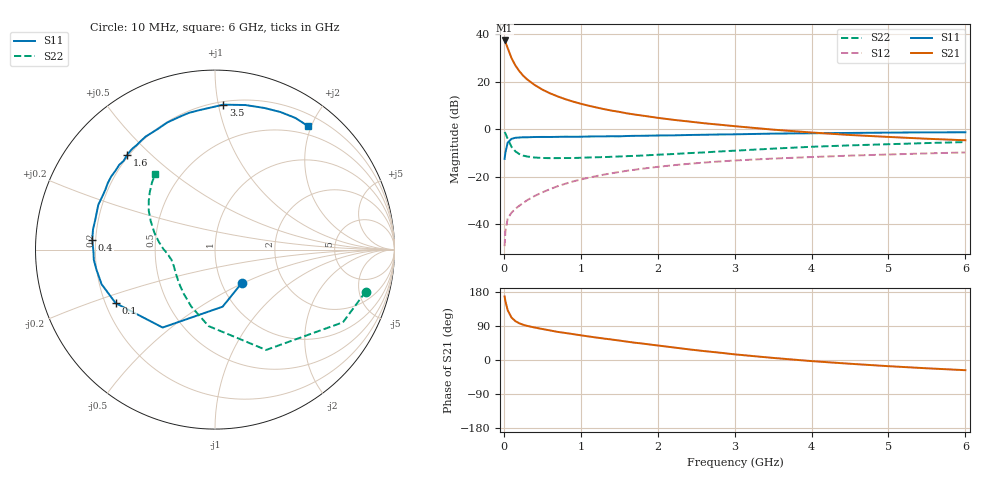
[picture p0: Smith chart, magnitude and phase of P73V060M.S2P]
! SIEMENS Small Signal Semiconductors
! BFP196
! Si NPN RF Bipolar Junction Transistor in SOT143
! VCE = 3 V  IC = 60 mA
! Common Emitter S-Parameters:  May  1996
# GHz  S  MA  R  50
!  f  S11  S21  S12  S22
! GHz  MAG  ANG  MAG  ANG  MAG  ANG  MAG  ANG
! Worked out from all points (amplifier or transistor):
!   36 points, 10 MHz to 6 GHz, reference 50 ohm
!   highest |S21| = 37.3 dB at 10 MHz (marker M1)
!   |S21| within 3 dB of that: start of sweep to 47.61 MHz
!   unconditionally stable (mu >= 1): 413.5 MHz to 4.553 GHz
!   at 250 MHz: K = 0.88, MSG = 26.8 dB, |S12| = -31.0 dB
!   at 1.4 GHz: K = 1.09, MAG = 11.4 dB, |S12| = -18.5 dB
!   at 6 GHz: K = 0.98, MSG = 2.6 dB, |S12| = -9.7 dB
!   S11 on the Smith chart (normalised r, x): 10 MHz: 1.24, -0.49; 100 MHz: 0.24, -0.24; 400 MHz: 0.19, +0.04; 1.6 GHz: 0.19, +0.42; 3.5 GHz: 0.22, +1.03; 6 GHz: 0.37, +1.95
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0.01  0.2386 -51.5  73.17 167.7  0.0035 78.8  0.8715 -15.6
0.02  0.3209 -82.4  67.9 155.5  0.0071 73.5  0.82 -29.6
0.05  0.5231 -123.9  50.6 131.3  0.0134 54.8  0.6275 -63.0
0.1  0.6288 -151.7  31.11 111.9  0.0177 50.1  0.4276 -94.8
0.15  0.6606 -163.0  21.84 102.6  0.0213 50.2  0.3428 -112.9
0.2  0.6698 -170.3  16.71 96.9  0.0247 54.6  0.302 -125.0
0.25  0.6777 -175.2  13.38 93.1  0.0281 56.8  0.2797 -134.2
0.3  0.6772 -178.9  11.24 90.2  0.0321 59.2  0.268 -140.1
0.4  0.6863 175.3  8.51 85.7  0.0397 62.2  0.2546 -149.4
0.5  0.6889 170.6  6.805 81.8  0.0472 63.7  0.249 -155.1
0.6  0.6874 166.4  5.68 78.0  0.0552 63.9  0.247 -159.0
0.7  0.6913 162.1  4.888 74.2  0.0636 64.2  0.2475 -162.1
0.9  0.6941 155.3  3.803 68.3  0.0801 62.8  0.2486 -166.7
1.1  0.703 148.2  3.127 62.2  0.0957 61.0  0.255 -169.8
1.3  0.7077 141.5  2.649 56.6  0.1113 58.4  0.26 -172.7
1.6  0.7206 132.7  2.155 48.5  0.1341 54.4  0.2721 -176.5
2.2  0.743 115.8  1.579 33.3  0.1753 45.4  0.3013 175.7
2.8  0.7757 100.8  1.247 19.5  0.21 36.5  0.341 166.5
3.5  0.8088 86.7  0.98 5.5  0.2419 26.5  0.3911 156.2
4.5  0.8358 70.7  0.757 -9.9  0.279 14.6  0.458 143.7
5.5  0.8594 58.6  0.631 -21.9  0.3108 3.7  0.5123 133.3
6  0.8617 53.0  0.586 -26.9  0.3255 -2.0  0.5375 128.2
